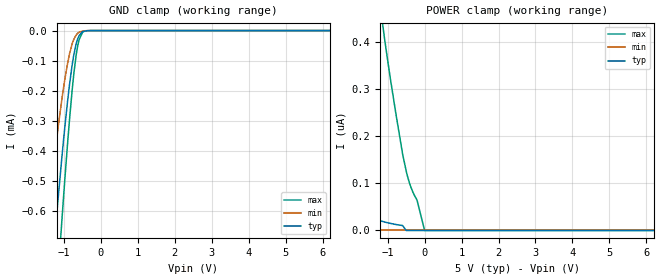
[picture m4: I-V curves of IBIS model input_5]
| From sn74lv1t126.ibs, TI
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|   input_5 Model
[Model]   input_5
Model_type   Input
Vinl = 0.8
Vinh = 2.02
|   typ   min   max
|   (nom PVT)   (fast PVT)   (slow PVT)
C_comp   5.160e-13   5.160e-13   5.189e-13
[Model spec]
|subparameter
Vinl   0.8   0.8   0.8
Vinh   2.02   2.02   2.1
| Where nom  PVT is Nominal Process, 5V, 40C
|   Fast PVT is Strong Process,  5.5V, -40C
|   Slow PVT is Weak Process,   4.5V, 140C
[Voltage Range]   5   4.5   5.5
|Junction Temperature
[Temperature Range]   40   140   -40
[Power Clamp Reference]   5   4.5   5.5
[GND Clamp Reference]   0   0   0
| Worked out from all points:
|   GND clamp passes 1 mA (typ) near -1.45 V on its own axis
[GND Clamp]
|   Voltage   I(typ)   I(min)   I(max)
-5V       -7.642mA   -5.851mA   -8.826mA
-1.56V    -1.167mA   -760.3uA   -1.575mA
-1.445V   -985.3uA   -627.1uA   -1.352mA
-1.229V   -660.5uA   -393.5uA   -943uA
-1.145V   -541uA     -309.8uA   -788.7uA
-1.044V   -407.1uA   -218.6uA   -611.9uA
-845mV    -176.2uA   -75.71uA   -291uA
-729.5mV  -79.1uA    -28.26uA   -141.3uA
-589mV    -16.65uA   -5.532uA   -30.24uA
-490mV    -3.771uA   -1.499uA   -5.673uA
-311mV    -190.2nA   -126.6nA   -176.1nA
10V       0A         0A         0A
[POWER Clamp]
|   Voltage   I(typ)   I(min)   I(max)
-5V       452.9nA    0A         5.583uA
-4.665V   376.9nA    0A         4.955uA
-3.74V    211nA      0A         3.36uA
-3.165V   138nA      0A         2.49uA
-2.228V   60.97nA    0A         1.33uA
-1.24V    21.51nA    0A         500.3nA
-1.084V   18nA       0A         406.9nA
-770.5mV  12.57nA    0A         244.2nA
-500mV    0A         0A         126.4nA
-207.5mV  0A         0A         64.94nA
-84.44fV  0A         0A         0A
10V       0A         0A         0A
